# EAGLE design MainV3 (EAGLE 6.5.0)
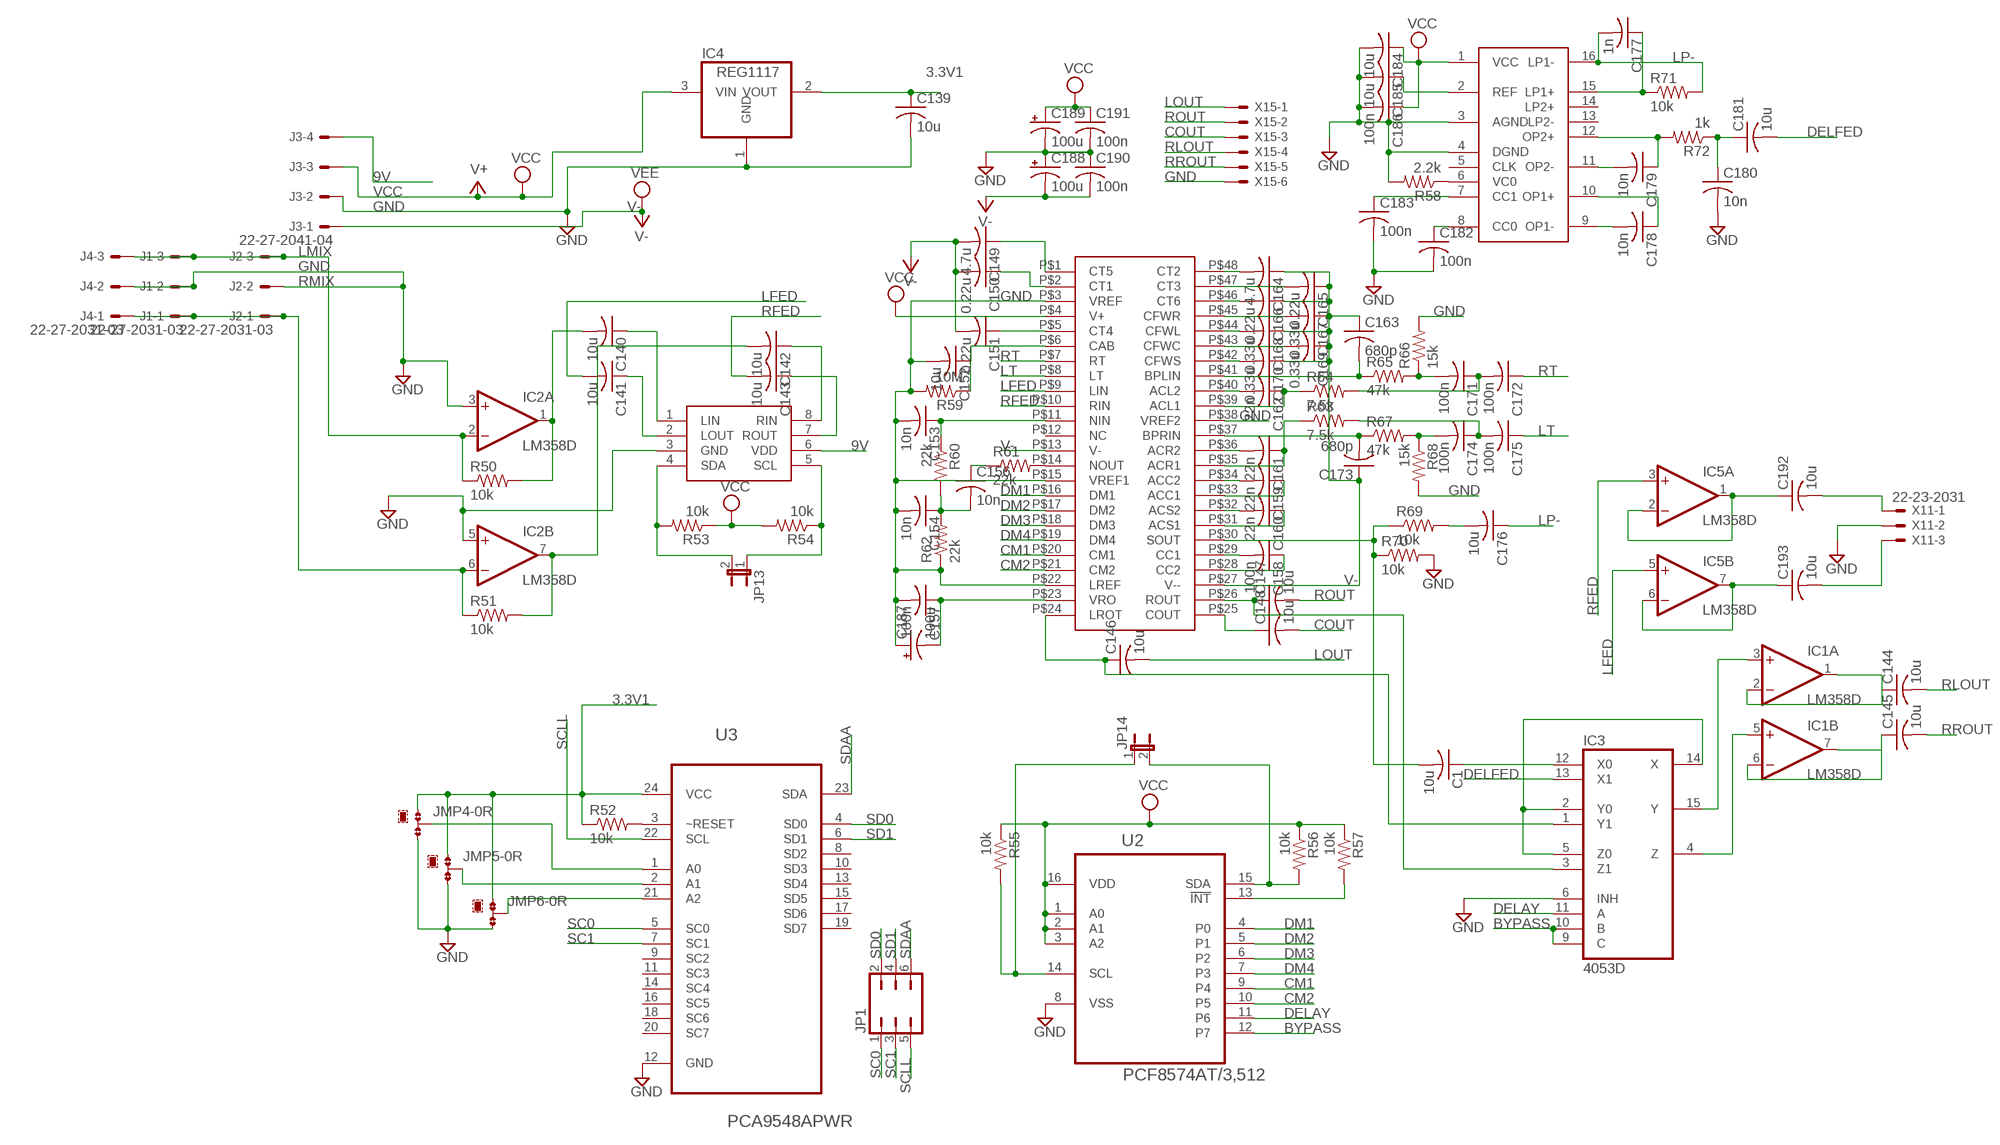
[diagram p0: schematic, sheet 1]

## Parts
C1  10u  C-USC1206  [C1206]
C139  10u  C-USC1206  [C1206]
C140  10u  C-USC1206  [C1206]
C141  10u  C-USC1206  [C1206]
C142  10u  C-USC1206  [C1206]
C143  10u  C-USC1206  [C1206]
C144  10u  C-USC1206  [C1206]
C145  10u  C-USC1206  [C1206]
C146  10u  C-USC1206  [C1206]
C147  10u  C-USC1206  [C1206]
C148  10u  C-USC1206  [C1206]
C149  4.7u  C-USC1206  [C1206]
C150  0.22u  C-USC1206  [C1206]
C151  0.22u  C-USC1206  [C1206]
C152  10u  C-USC1206  [C1206]
C153  10n  C-USC1206  [C1206]
C154  10n  C-USC1206  [C1206]
C156  10n  C-USC1206  [C1206]
C157  100n  C-USC1206  [C1206]
C158  100n  C-USC1206  [C1206]
C159  22n  C-USC1206  [C1206]
C160  22n  C-USC1206  [C1206]
C161  22n  C-USC1206  [C1206]
C162  22n  C-USC1206  [C1206]
C163  680p  C-USC1206  [C1206]
C164  4.7u  C-USC1206  [C1206]
C165  0.22u  C-USC1206  [C1206]
C166  0.22u  C-USC1206  [C1206]
C167  0.33u  C-USC1206  [C1206]
C168  0.33u  C-USC1206  [C1206]
C169  0.33u  C-USC1206  [C1206]
C170  0.33u  C-USC1206  [C1206]
C171  100n  C-USC1206  [C1206]
C172  100n  C-USC1206  [C1206]
C173  680p  C-USC1206  [C1206]
C174  100n  C-USC1206  [C1206]
C175  100n  C-USC1206  [C1206]
C176  10u  C-USC1206  [C1206]
C177  1n  C-USC1206  [C1206]
C178  10n  C-USC1206  [C1206]
C179  10n  C-USC1206  [C1206]
C180  10n  C-USC1206  [C1206]
C181  10u  C-USC1206  [C1206]
C182  100n  C-USC1206  [C1206]
C183  100n  C-USC1206  [C1206]
C184  10u  C-USC1206  [C1206]
C185  10u  C-USC1206  [C1206]
C186  100n  C-USC1206  [C1206]
C187  100u  CPOL-USE2-5  [E2-5]
C188  100u  CPOL-USE2-5  [E2-5]
C189  100u  CPOL-USE2-5  [E2-5]
C190  100n  C-USC1206  [C1206]
C191  100n  C-USC1206  [C1206]
C192  10u  C-USC1206  [C1206]
C193  10u  C-USC1206  [C1206]
IC1  LM358D  [SO08]
IC2  LM358D  [SO08]
IC3  4053D  [SO16]
IC4  REG1117  [SOT223]
IC5  LM358D  [SO08]
J1  22-27-2031-03  [6410-03]
J2  22-27-2031-03  [6410-03]
J3  22-27-2041-04  [6410-04]
J4  22-27-2031-03  [6410-03]
JMP4  0R-JUMPB  [B0R-JMP]
JMP5  0R-JUMPB  [B0R-JMP]
JMP6  0R-JUMPB  [B0R-JMP]
JP1  JP3Q  [JP3Q]
JP13  JP1E  [JP1]
JP14  JP1E  [JP1]
R50  10k  R-US_R1206  [R1206]
R51  10k  R-US_R1206  [R1206]
R52  10k  R-US_R1206  [R1206]
R53  10k  R-US_R1206  [R1206]
R54  10k  R-US_R1206  [R1206]
R55  10k  R-US_R1206  [R1206]
R56  10k  R-US_R1206  [R1206]
R57  10k  R-US_R1206  [R1206]
R58  2.2k  R-US_R1206  [R1206]
R59  10M  R-US_R1206  [R1206]
R60  22k  R-US_R1206  [R1206]
R61  22k  R-US_R1206  [R1206]
R62  22k  R-US_R1206  [R1206]
R63  7.5k  R-US_R1206  [R1206]
R64  7.5k  R-US_R1206  [R1206]
R65  47k  R-US_R1206  [R1206]
R66  15k  R-US_R1206  [R1206]
R67  47k  R-US_R1206  [R1206]
R68  15k  R-US_R1206  [R1206]
R69  10k  R-US_R1206  [R1206]
R70  10k  R-US_R1206  [R1206]
R71  10k  R-US_R1206  [R1206]
R72  1k  R-US_R1206  [R1206]
U2  PCF8574AT/3,512  [SOIC127P1032X265-16N]
U3  PCA9548APWR  [SOP65P640X120-24N]
U$9  SSM2126  [DIP48]
U$10  PT2257  [SO08]
U$11  PT2399  [DIL16]
X11  22-23-2031  [22-23-2031]
X15  22-23-2061  [22-23-2061]

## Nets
3.3V1: C139.1 IC4.2(VOUT) JMP4.1 JMP5.1 JMP6.1 R52.1 U3.24(VCC)
9V: J3.4 U$10.6(VDD)
BYPASS: IC3.9(C) IC3.10(B) U2.12(P7)
CM1: U2.9(P4) U$9.P$20(CM1)
CM2: U2.10(P5) U$9.P$21(CM2)
COUT: C148.2 X15.3
DELAY: IC3.11(A) U2.11(P6)
DELFED: C181.2 IC3.13(X1)
DM1: U2.4(P0) U$9.P$16(DM1)
DM2: U2.5(P1) U$9.P$17(DM2)
DM3: U2.6(P2) U$9.P$18(DM3)
DM4: U2.7(P3) U$9.P$19(DM4)
GND: C139.2 C152.2 C153.2 C154.2 C157.2 C180.2 C182.2 C183.2 C184.2 C185.2 C186.2 C187.+ C188.+ C189.- C190.1 C191.2 IC2.3(A:+IN) IC2.5(B:+IN) IC3.6(INH) IC4.1(GND) J1.2 J2.2 J3.2 J4.2 JMP4.3 JMP5.3 JMP6.3 R58.2 R59.2 R62.1 R66.2 R68.2 R70.2 U2.8(VSS) U3.12(GND) U$9.P$3(VREF) U$9.P$15(VREF1) U$9.P$22(LREF) U$9.P$38(VREF2) U$10.3(GND) U$11.3(AGND) U$11.4(DGND) X11.2 X15.6
LFED: C141.2 IC5.5(B:+IN) U$9.P$9(LIN)
LMIX: IC2.2(A:-IN) J1.3 J2.3 J4.3 R50.1
LOUT: C146.2 X15.1
LP-: C176.1 C177.2 R71.2 U$11.16(LP1-)
LT: C175.1 U$9.P$8(LT)
N$1: C1.1 IC3.12(X0)
N$2: C146.1 IC3.1(Y1) U$9.P$24(LROT)
N$3: C147.1 IC3.3(Z1) U$9.P$26(ROUT)
N$4: C144.1 IC1.1(A:OUT) IC1.2(A:-IN)
N$5: C145.1 IC1.6(B:-IN) IC1.7(B:OUT)
N$7: IC1.3(A:+IN) IC3.15(Y)
N$8: IC1.5(B:+IN) IC3.4(Z)
N$241: C140.2 IC2.1(A:OUT) R50.2
N$242: C192.1 IC5.1(A:OUT) IC5.2(A:-IN)
N$243: C193.1 IC5.6(B:-IN) IC5.7(B:OUT)
N$244: C142.2 IC2.7(B:OUT) R51.2
N$245: C140.1 U$10.1(LIN)
N$246: C142.1 U$10.8(RIN)
N$247: C141.1 U$10.2(LOUT)
N$248: C143.1 U$10.7(ROUT)
N$249: R52.2 U3.3(~RESET)
N$257: C192.2 X11.1
N$258: JMP5.2 U3.2(A1)
N$260: JMP6.2 U3.21(A2)
N$261: JMP4.2 U3.1(A0)
N$262: IC3.2(Y0) IC3.5(Z0) IC3.14(X)
N$263: R57.2 U2.13(!INT)
N$268: C148.1 U$9.P$25(COUT)
N$269: R58.1 U$11.6(VC0)
N$270: C149.1 U$9.P$1(CT5)
N$271: C150.1 U$9.P$2(CT1)
N$272: C151.1 U$9.P$5(CT4)
N$273: C152.1 R59.1 U$9.P$6(CAB)
N$274: R61.2 U$9.P$14(NOUT)
N$278: C153.1 R60.1 U$9.P$11(NIN)
N$279: C193.2 X11.3
N$281: C154.1 C156.2 R60.2 R62.2
N$282: C156.1 R61.1
N$283: C157.1 C187.- U$9.P$23(VRO)
N$284: C158.2 U$9.P$29(CC1)
N$285: C158.1 U$9.P$28(CC2)
N$286: C160.1 U$9.P$31(ACS1)
N$287: C160.2 U$9.P$32(ACS2)
N$289: C159.1 U$9.P$33(ACC1)
N$290: C159.2 U$9.P$34(ACC2)
N$291: C161.1 R63.1 U$9.P$35(ACR1)
N$292: C161.2 U$9.P$36(ACR2)
N$293: C162.2 U$9.P$40(ACL2)
N$294: C162.1 R64.1 U$9.P$39(ACL1)
N$295: C163.2 R65.1 U$9.P$41(BPLIN)
N$296: C166.2 U$9.P$46(CT6)
N$297: C170.2 U$9.P$42(CFWS)
N$298: C169.2 U$9.P$43(CFWC)
N$299: C168.2 U$9.P$44(CFWL)
N$300: C167.2 U$9.P$45(CFWR)
N$301: C165.2 U$9.P$47(CT3)
N$302: C164.2 U$9.P$48(CT2)
N$303: C171.2 R65.2 R66.1
N$304: C171.1 C172.2 R64.2
N$305: C173.2 R67.1 U$9.P$37(BPRIN)
N$306: C174.2 R67.2 R68.1
N$307: C174.1 C175.2 R63.2
N$308: C176.2 R69.2
N$309: C177.1 R71.1 U$11.15(LP1+)
N$310: C178.2 U$11.9(OP1-)
N$311: C179.2 U$11.11(OP2-)
N$312: C178.1 U$11.10(OP1+)
N$313: C179.1 R72.2 U$11.12(OP2+)
N$314: C180.1 C181.1 R72.1
N$315: C183.1 U$11.7(CC1)
N$316: C182.1 U$11.8(CC0)
N$317: C185.1 U$11.2(REF)
N$318: JP13.2 R53.2 U$10.4(SDA)
N$319: JP13.1 R54.1 U$10.5(SCL)
N$320: JP14.2 R56.2 U2.15(SDA)
N$321: JP14.1 R55.2 U2.14(SCL)
RFED: C143.2 IC5.3(A:+IN) U$9.P$10(RIN)
RLOUT: C144.2 X15.4
RMIX: IC2.6(B:-IN) J1.1 J2.1 J4.1 R51.1
ROUT: C147.2 X15.2
RROUT: C145.2 X15.5
RT: C172.1 U$9.P$7(RT)
SC0: JP1.1 U3.5(SC0)
SC1: JP1.3 U3.7(SC1)
SCLL: JP1.5 U3.22(SCL)
SD0: JP1.2 U3.4(SD0)
SD1: JP1.4 U3.6(SD1)
SDAA: JP1.6 U3.23(SDA)
SFED: C1.2 R69.1 R70.1 U$9.P$30(SOUT)
V-: C149.2 C150.2 C151.2 C163.1 C164.1 C165.1 C166.1 C167.1 C168.1 C169.1 C170.1 C173.1 C188.- C190.2 J3.1 U$9.P$13(V-) U$9.P$27(V--) ; supply symbol labelled VEE
VCC: C184.1 C186.1 C189.+ C191.1 IC4.3(VIN) J3.3 R53.1 R54.2 R55.1 R56.1 R57.1 U2.1(A0) U2.2(A1) U2.3(A2) U2.16(VDD) U$9.P$4(V+) U$11.1(VCC) ; supply symbol labelled V+
Unconnected: U3.8(SD2) U3.9(SC2) U3.10(SD3) U3.11(SC3) U3.13(SD4) U3.14(SC4) U3.15(SD5) U3.16(SC5) U3.17(SD6) U3.18(SC6) U3.19(SD7) U3.20(SC7) U$9.P$12(NC) U$11.5(CLK) U$11.13(LP2-) U$11.14(LP2+)

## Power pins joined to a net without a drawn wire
GND: IC3.8(GND)
V+: IC2.8(P:V+)
V-: IC1.4(P:V-) IC2.4(P:V-) IC3.7(VEE) IC5.4(P:V-)
VCC: IC1.8(P:V+) IC3.16(VCC) IC5.8(P:V+)

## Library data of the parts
C1 C139-C154 C156-C186 C190-C193 = adafruit:C-US: CAPACITOR, American symbol
C187-C189 = adafruit:CPOL-US: POLARIZED CAPACITOR, American symbol
IC1 IC2 IC5 = linear:LM358: OP AMP also LM158; LM258; LM2904 Source: http://cache.national.com/ds/LM/LM158.pdf
IC3 = 40xx:4053: Triple 2-channel ANALOG MULTIPLEXER
IC4 = burr-brown:REG1117: 800mA and 1A Low Dropout (LDO) Positive Regulator 1.8V, 2.5V, 2.85V, 3.3V, 5V, and Adj; MPN: REG1117; OC_FARNELL: 1097566; OC_NEWARK: 14P6981
J1 J2 J4 = con-molex:22-?-03: CONNECTOR wire to board 2.54 mm (.1 inch) pitch header; OC_FARNELL: unknown; OC_NEWARK: unknown
J3 = con-molex:22-?-04: CONNECTOR wire to board 2.54 mm (.1 inch) pitch header; OC_FARNELL: unknown; OC_NEWARK: unknown
JMP4-JMP6 = jump-0r-smd:0R-JUMP: SMD 0R 0805 Jumper
JP1 = jumper:JP3Q: JUMPER
JP13 JP14 = jumper:JP1E: JUMPER
R50-R72 = adafruit:R-US_: RESISTOR, American symbol
U2 = PCF8574A:PCF8574AT/3,512: IC, I/O EXPANDER, 8BIT, 16SOIC; MPN: PCF8574AT/3,512; OC_FARNELL: 2101302; OC_NEWARK: 70R6866; PACKAGE: SOIC-16; SUPPLIER: NXP
U3 = PCA9548A:PCA9548APWR: 8-CHANNEL I2C SWITCH WITH RESET; MPN: PCA9548APWR False; OC_FARNELL: 1607855; OC_NEWARK: 22M1602; PACKAGE: TSSOP-24; SUPPLIER: Texas Instruments
U$9 = adafruit:SSM2126
U$10 = adafruit:PT2257
U$11 = adafruit:PT2399
X11 = con-molex:22-23-2031: .100" (2.54mm) Center Header - 3 Pin; MF: MOLEX; MPN: 22-23-2031; OC_FARNELL: 1462950; OC_NEWARK: 30C0862
X15 = con-molex:22-23-2061: .100" (2.54mm) Center Header - 6 Pin; MF: MOLEX; MPN: 22-23-2061; OC_FARNELL: 1462922; OC_NEWARK: 27C1933

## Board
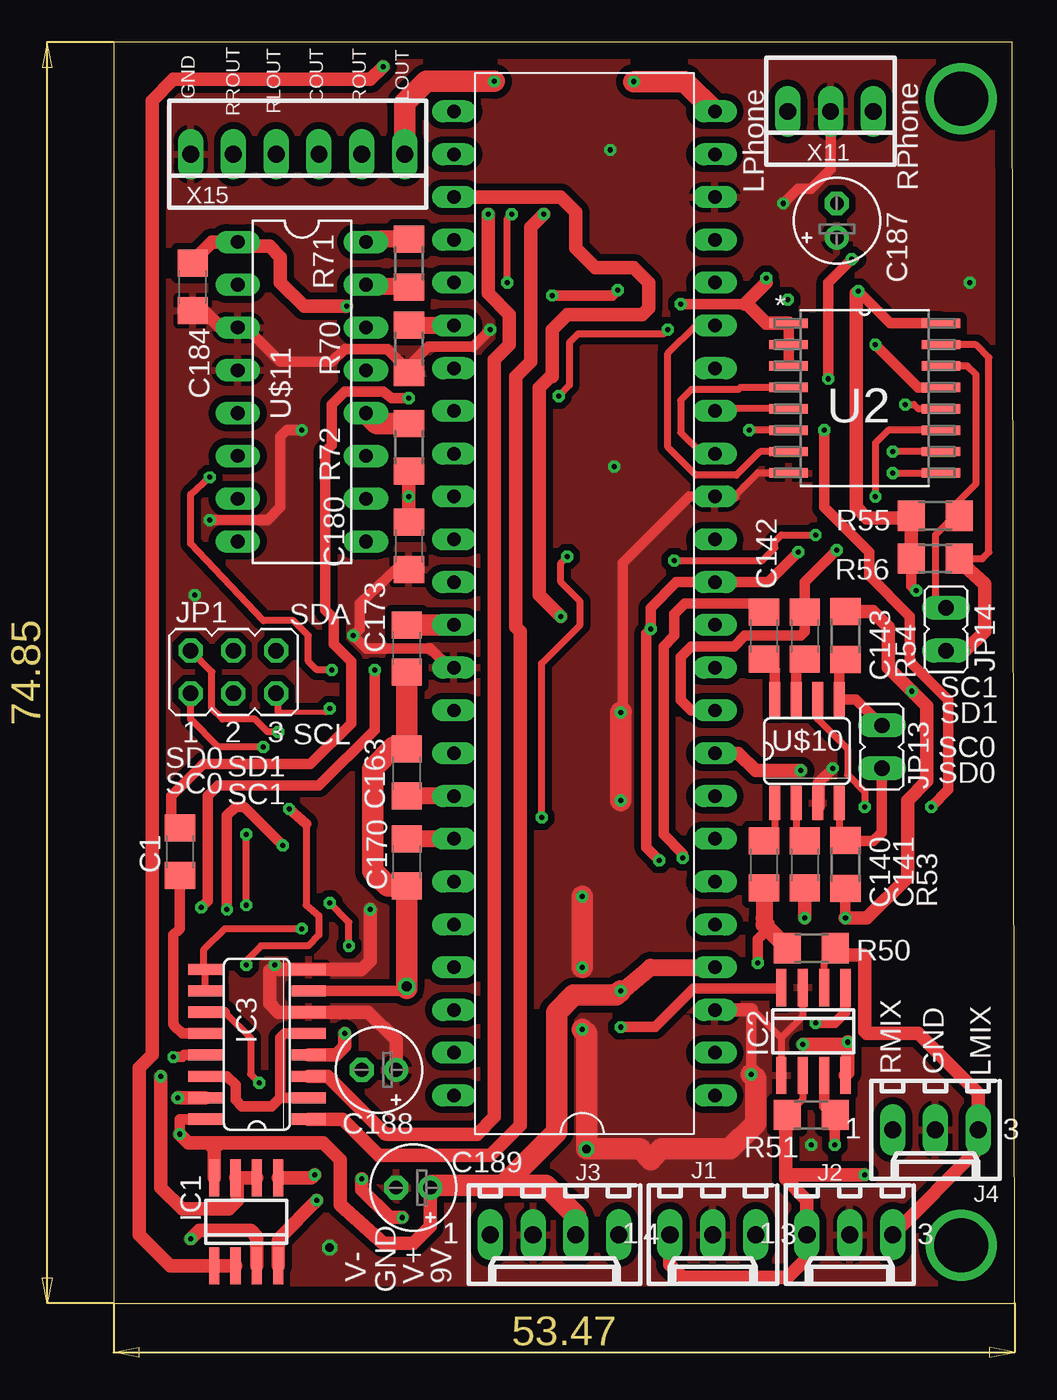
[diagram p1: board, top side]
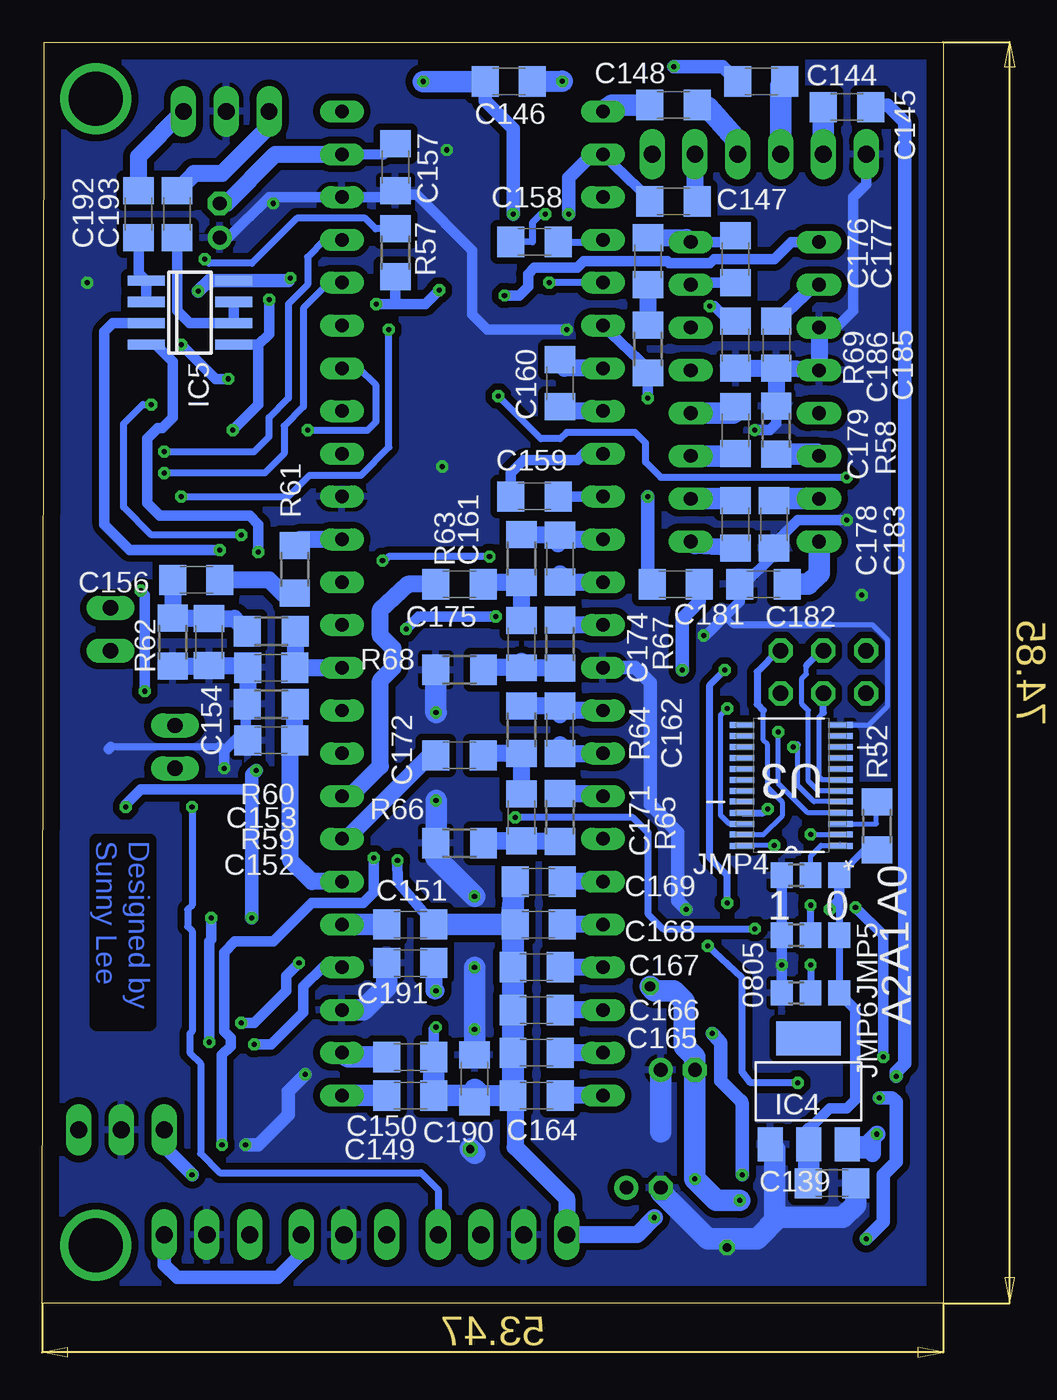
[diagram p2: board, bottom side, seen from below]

Size 57.71 x 78.08 mm. Coordinates in mm from the lower left corner, seen from the top.
Outline: 4.24,3.22 57.71,3.22 57.58,78.08 4.24,78.08 4.24,3.22
Copper layers (1*16): Top 0.035mm / dielectric 1.5mm / Bottom 0.035mm
Design rules "default *": minimum track width 10mil, minimum drill 0.3mm, track to track 6mil, track to pad 6mil, pad to pad 6mil, via to via 6mil, smd to smd 6mil, copper to edge 40mil, drill to drill 8mil, minimum pad ring 10mil, minimum via ring 8mil, stop-mask expansion 4mil, vias tented up to drill 0mil, thermal gap 10mil

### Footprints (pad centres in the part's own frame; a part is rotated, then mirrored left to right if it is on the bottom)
C1206 = smd 1.6 x 1.8: 1 -1.4,0; 2 1.4,0
E2-5 = drill 0.813 pad 1.422: + -1.016,0 | drill 0.813 pad 1.422 octagon: - 1.016,0
SO08 = smd 0.6 x 2.2: 1 -1.905,-2.6; 2 -0.635,-2.6; 3 0.635,-2.6; 4 1.905,-2.6; 5 1.905,2.6; 6 0.635,2.6; 7 -0.635,2.6; 8 -1.905,2.6
SO16 = smd 0.66 x 2.032: 1 -4.445,-3.073; 2 -3.175,-3.073; 3 -1.905,-3.073; 4 -0.635,-3.073; 5 0.635,-3.073; 6 1.905,-3.073; 7 3.175,-3.073; 8 4.445,-3.073; 9 4.445,3.073; 10 3.175,3.073; 11 1.905,3.073; 12 0.635,3.073; 13 -0.635,3.073; 14 -1.905,3.073; 15 -3.175,3.073; 16 -4.445,3.073
SOT223 = smd 1.499 x 2.007: 1 -2.261,-3.15; 2 0.025,-3.15; 3 2.311,-3.15 | smd 3.81 x 2.007: 4 0,3.15
6410-03 = drill 1.016 long: 1 2.54,0; 2 0,0; 3 -2.54,0
6410-04 = drill 1.016 long: 1 3.81,0; 2 1.27,0; 3 -1.27,0; 4 -3.81,0
B0R-JMP = smd 1.5 x 1.3: 1 0,1.7; 2 0,0; 3 0,-1.7
JP3Q = drill 0.914 octagon: 1 -2.54,-1.27; 2 -2.54,1.27; 3 0,-1.27; 4 0,1.27; 5 2.54,-1.27; 6 2.54,1.27
JP1 = drill 0.914 long: 1 0,-1.27; 2 0,1.27
R1206 = smd 1.6 x 1.803: 1 -1.422,0; 2 1.422,0
SOIC127P1032X265-16N = smd 2.286 x 0.559: 1 -4.521,4.445; 2 -4.521,3.175; 3 -4.521,1.905; 4 -4.521,0.635; 5 -4.521,-0.635; 6 -4.521,-1.905; 7 -4.521,-3.175; 8 -4.521,-4.445; 9 4.521,-4.445; 10 4.521,-3.175; 11 4.521,-1.905; 12 4.521,-0.635; 13 4.521,0.635; 14 4.521,1.905; 15 4.521,3.175; 16 4.521,4.445
SOP65P640X120-24N = smd 1.473 x 0.356: 1 -2.921,3.581; 2 -2.921,2.921; 3 -2.921,2.286; 4 -2.921,1.626; 5 -2.921,0.965; 6 -2.921,0.33; 7 -2.921,-0.33; 8 -2.921,-0.965; 9 -2.921,-1.626; 10 -2.921,-2.286; 11 -2.921,-2.921; 12 -2.921,-3.581; 13 2.921,-3.581; 14 2.921,-2.921; 15 2.921,-2.286; 16 2.921,-1.626; 17 2.921,-0.965; 18 2.921,-0.33; 19 2.921,0.33; 20 2.921,0.965; 21 2.921,1.626; 22 2.921,2.286; 23 2.921,2.921; 24 2.921,3.581
DIP48 = drill 0.8 long: P$1 -29.21,-8.89; P$2 -26.67,-8.89; P$3 -24.13,-8.89; P$4 -21.59,-8.89; P$5 -19.05,-8.89; P$6 -16.51,-8.89; P$7 -13.97,-8.89; P$8 -11.43,-8.89; P$9 -8.89,-8.89; P$10 -6.35,-8.89; P$11 -3.81,-8.89; P$12 -1.27,-8.89; P$13 1.27,-8.89; P$14 3.81,-8.89; P$15 6.35,-8.89; P$16 8.89,-8.89; P$17 11.43,-8.89; P$18 13.97,-8.89; P$19 16.51,-8.89; P$20 19.05,-8.89; P$21 21.59,-8.89; P$22 24.13,-8.89; P$23 26.67,-8.89; P$24 29.21,-8.89; P$25 29.21,6.604; P$26 26.67,6.604; P$27 24.13,6.604; P$28 21.59,6.604; P$29 19.05,6.604; P$30 16.51,6.604; P$31 13.97,6.604; P$32 11.43,6.604; P$33 8.89,6.604; P$34 6.35,6.604; P$35 3.81,6.604; P$36 1.27,6.604; P$37 -1.27,6.604; P$38 -3.81,6.604; P$39 -6.35,6.604; P$40 -8.89,6.604; P$41 -11.43,6.604; P$42 -13.97,6.604; P$43 -16.51,6.604; P$44 -19.05,6.604; P$45 -21.59,6.604; P$46 -24.13,6.604; P$47 -26.67,6.604; P$48 -29.21,6.604
SO08' = smd 0.66 x 2.032: 1 -1.905,-3.073; 2 -0.635,-3.073; 3 0.635,-3.073; 4 1.905,-3.073; 5 1.905,3.073; 6 0.635,3.073; 7 -0.635,3.073; 8 -1.905,3.073
DIL16 = drill 0.813 long: 1 -8.89,-3.81; 2 -6.35,-3.81; 3 -3.81,-3.81; 4 -1.27,-3.81; 5 1.27,-3.81; 6 3.81,-3.81; 7 6.35,-3.81; 8 8.89,-3.81; 9 8.89,3.81; 10 6.35,3.81; 11 3.81,3.81; 12 1.27,3.81; 13 -1.27,3.81; 14 -3.81,3.81; 15 -6.35,3.81; 16 -8.89,3.81
22-23-2031 = drill 1 long: 1 -2.54,0; 2 0,0; 3 2.54,0
22-23-2061 = drill 1 long: 1 -6.35,0; 2 -3.81,0; 3 -1.27,0; 4 1.27,0; 5 3.81,0; 6 6.35,0

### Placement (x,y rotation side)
C1  8.17,30.02 90 top
C139  10.84,10.33 0 bottom
C140  42.84,29.26 270 top
C141  45.26,29.26 270 top
C142  42.84,42.84 90 top
C143  45.26,42.84 90 top
C144  15.03,75.74 0 bottom
C145  9.95,74.21 180 bottom
C146  30.02,75.74 0 bottom
C147  20.24,68.63 0 bottom
C148  20.24,74.34 0 bottom
C149  35.86,15.54 0 bottom
C150  35.86,17.83 0 bottom
C151  35.86,25.7 0 bottom
C152  44.12,36.62 180 bottom
C153  44.12,40.94 180 bottom
C154  47.8,42.46 270 bottom
C156  48.56,46.15 180 bottom
C157  36.75,70.66 270 bottom
C158  28.49,66.21 180 bottom
C159  28.49,51.1 0 bottom
C160  26.97,57.83 270 bottom
C161  26.97,47.42 270 bottom
C162  26.97,37.26 270 bottom
C163  21.64,34.72 270 top
C164  28.37,15.54 0 bottom
C165  28.37,18.08 0 bottom
C166  28.37,20.62 0 bottom
C167  28.37,23.16 0 bottom
C168  28.24,25.7 0 bottom
C169  28.24,28.24 0 bottom
C170  21.64,29.38 90 top
C171  29.26,32.05 270 bottom
C172  32.94,35.73 0 bottom
C173  21.64,42.08 90 top
C174  29.26,42.34 270 bottom
C175  32.94,45.89 0 bottom
C176  21.76,65.07 270 bottom
C177  16.56,65.2 90 bottom
C178  16.56,49.45 270 bottom
C179  16.56,55.04 270 bottom
C180  21.76,48.18 270 top
C181  20.11,45.89 0 bottom
C182  14.9,45.89 180 bottom
C183  14.27,49.45 270 bottom
C184  8.94,63.55 270 top
C185  14.14,60.12 270 bottom
C186  16.56,60.12 270 bottom
C187  47.16,67.48 90 top
C188  19.98,17.06 180 top
C189  22.02,10.08 180 top
C190  32.05,16.56 270 bottom
C191  35.86,23.41 180 bottom
C192  51.99,67.86 90 bottom
C193  49.7,67.86 90 bottom
IC1  12.11,8.05 0 top
IC2  45.77,19.35 180 top
IC3  12.75,18.59 90 top
IC4  12.24,15.79 0 bottom
IC5  48.94,62.02 270 bottom
J1  39.8,7.29 180 top
J2  47.92,7.29 180 top
J3  30.4,7.29 180 top
J4  53.01,13.51 180 top
JMP4  12.11,28.62 270 bottom
JMP5  12.11,25.07 270 bottom
JMP6  12.11,21.64 270 bottom
JP1  11.35,40.69 0 top
JP13  49.83,36.24 180 top
JP14  53.64,43.23 180 top
R50  45.64,24.3 180 top
R51  45.64,14.4 0 top
R52  8.17,31.54 90 bottom
R53  47.67,29.26 90 top
R54  47.67,42.84 90 top
R55  53.01,49.96 0 top
R56  53.01,47.42 0 top
R57  36.75,65.58 90 bottom
R58  14.14,55.04 90 bottom
R59  44.12,38.78 180 bottom
R60  44.12,43.1 180 bottom
R61  42.72,46.78 90 bottom
R62  49.96,42.46 90 bottom
R63  29.26,47.42 270 bottom
R64  29.26,37.26 270 bottom
R65  26.97,32.05 270 bottom
R66  32.94,30.53 180 bottom
R67  26.97,42.34 270 bottom
R68  32.94,40.81 180 bottom
R69  21.76,59.86 90 bottom
R70  21.76,59.86 270 top
R71  21.76,64.94 90 top
R72  21.76,54.02 90 top
U2  48.81,56.94 0 top
U3  13.25,33.95 180 bottom
U$9  31.03,44.75 90 top
U$10  PT2257  [SO08']  45.38,35.99 0 top
U$11  15.41,57.32 270 top
X11  46.78,73.96 180 top
X15  15.16,71.42 180 top

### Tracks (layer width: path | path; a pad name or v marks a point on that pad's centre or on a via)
3.3V1  (via drill 0.3)
  Top 0.61: v10.97,26.59 10.97,32.18 11.48,32.69 11.98,32.69 v14.27,30.4
  Bottom 0.305: v14.27,30.4 16.15,30.4 U3.24
  Bottom 0.406: 10.41,27.15 JMP5.1 JMP6.1 | R52.1 8.91,30.12 JMP4.1
  Bottom 0.61: JMP6.1 9.44,20.67 9.44,15.29 9.95,14.78 10.97,14.78 12.21,13.53 | JMP4.1 10.41,27.15 v10.97,26.59
  Bottom 0.813: 12.21,13.53 IC4.2
  Bottom 1.27: IC4.2 12.21,10.36 C139.1
9V  (via drill 0.3)
  Top 0.406: U$10.6 46.02,37.89 47.8,36.11 47.8,34.59 48.81,33.57 v48.81,32.69
  Bottom 0.406: v48.81,32.69 48.81,26.84 49.07,26.59 49.07,25.57 48.81,25.32 48.81,19.35 48.94,19.22 48.94,18.08 48.31,17.45 48.31,12.11 47.16,10.97 35.23,10.97 34.21,9.95 J3.4
BYPASS  (via drill 0.3)
  Top 0.406: IC3.10 IC3.9 | v15.41,25.45 10.84,25.45 9.57,24.18 9.57,23.14 | v29.64,32.05 29.64,41.19 31.92,43.48 31.92,44.88 30.78,46.02 30.78,47.16 v31.16,47.54 | v37.51,47.29 42.72,47.29 43.48,48.05 43.48,48.43 43.86,48.81 v45.89,48.81 | v51.23,56.56 51.73,56.56 51.99,56.31 U2.12
  Top 0.61: 9.57,23.14 IC3.9
  Bottom 0.406: v15.41,25.45 20.87,25.45 21.76,26.34 21.76,31.16 22.65,32.05 v29.64,32.05 | v31.16,47.54 37.13,47.54 37.38,47.29 v37.51,47.29 | v51.23,56.56 51.73,56.56 52.88,55.42 52.88,50.47 51.23,48.81 v45.89,48.81
CM1  (via drill 0.3)
  Top 0.406: v50.46,52.5 U2.9
  Bottom 0.406: U$9.P$20 40.69,63.8 42.21,62.28 42.21,56.43 43.35,55.29 43.35,53.64 44.5,52.5 v50.46,52.5
CM2  (via drill 0.3)
  Top 0.406: U2.10 v50.46,53.77
  Bottom 0.406: v50.46,53.77 45.13,53.77 44.24,54.66 44.24,55.8 43.1,56.94 43.1,62.53 41.96,63.67 41.96,65.32 40.94,66.34 U$9.P$21
COUT
  Bottom 1.27: C148.2 18.21,74.21 16.43,72.18 X15.3
DELAY  (via drill 0.3)
  Top 0.406: 10.84,20.49 12.36,18.97 12.36,16.81 v12.87,16.3 | v18.21,24.43 18.21,25.83 v17.06,26.97 | v17.19,40.81 16.3,40.81 15.79,41.32 15.79,42.84 14.9,43.73 13.13,43.73 8.81,48.31 8.81,51.23 v9.95,52.24 | U2.11 50.21,55.04 49.45,54.28 v49.45,51.1 | v37.13,61.01 36.88,60.75 31.8,60.75 31.29,60.24 31.29,57.7 v30.65,57.07
  Top 0.61: IC3.11 10.84,20.49
  Bottom 0.406: v9.95,52.24 21,52.24 21.89,53.13 21.89,54.28 22.52,54.91 26.59,54.91 26.97,54.53 28.11,54.53 v30.65,57.07 | v12.87,16.3 15.67,16.3 16.17,16.94 16.17,22.52 v18.21,24.43 | v17.06,26.97 17.06,28.62 18.08,29.64 18.08,39.92 v17.19,40.81 | v49.45,51.1 43.1,51.1 41.83,52.37 38.78,52.37 37.13,54.02 v37.13,61.01
DELFED  (via drill 0.3)
  Top 0.61: v19.73,40.81 19.73,37.26 16.43,33.95 10.46,33.95 9.82,33.32 9.82,27.1 v9.44,26.72 | v7.79,17.83 8.3,17.83 8.43,17.95 IC3.13
  Bottom 0.61: C181.2 18.71,45 | v9.44,26.72 7.79,25.07 v7.79,17.83
  Bottom 0.813: 18.71,45 18.71,44.88 19.73,43.86 v19.73,40.81
DM1
  Top 0.406: U2.4 41.45,57.58 41.32,57.45 38.53,57.45 37.89,56.81 37.89,54.91 39.16,53.64 U$9.P$16
DM2
  Top 0.406: U2.5 40.05,56.31 U$9.P$17
DM3  (via drill 0.3)
  Top 0.406: U2.6 v41.96,55.04
  Bottom 0.406: v41.96,55.04 38.4,55.04 37.89,55.55 37.89,57.7 38.91,58.72 U$9.P$18
DM4
  Top 0.406: U2.7 42.59,53.77 41.19,52.37 38.78,52.37 37.13,54.02 37.13,59.61 38.78,61.26 U$9.P$19
GND  (via drill 0.3, 0.5)
  Top 0.406: U$10.3 46.02,32.81 46.15,32.69 | IC2.3 45.13,20.24 43.86,18.97 | 43.86,18.97 IC2.5 | 42.08,20.62 42.21,20.62 43.86,18.97 | U2.8 42.46,52.5 41.07,51.1
  Top 0.61: U$10.3 46.02,34.08 v46.91,34.97 46.15,34.21 46.15,32.69 | v42.08,16.81 42.08,20.62 | 41.07,51.1 U$9.P$15 38.4,51.1 34.46,47.16 34.46,38.4 v34.34,38.27 | v26.59,61.01 25.57,59.99 22.91,59.99 21.76,58.85 R70.2 21.76,58.59 20.49,59.86 17.95,59.86 17.19,59.1 14.14,59.1 12.11,61.13 | 13.51,22.98 v13.81,23.29 | IC3.8 15.29,23.03 | C180.2 21,46.78 18.84,44.75 18.84,43.23 v18.46,42.84 19.22,42.08 23.03,42.08 24.18,40.94 U$9.P$38 | v15.41,55.04 14.52,55.04 14.14,54.66 14.14,50.47 13.38,49.7 v9.95,49.7 | X11.2 46.78,70.53 45.64,69.39 44.88,69.39 v43.99,68.5
  Top 0.813: U$9.P$3 42.08,20.62 | C184.2 9.57,62.15 10.59,61.13 U$11.3 | 13.51,22.98 13.51,21 14.02,20.49 IC3.6 19.35,20.49 21,18.84 C188.+ | v13.81,23.29 14.06,23.03 15.29,23.03 18.97,23.03 19.48,23.54 v19.48,26.59
  Top 1.016: 12.11,61.13 U$11.3
  Top 1.27: v32.05,27.35 v32.05,23.16 | v34.34,33.07 v34.34,38.27 34.36,38.3 | v32.05,19.48 32.3,19.22 v32.3,12.37 35.48,12.37 36.11,11.73 36.75,12.37 40.81,12.37 42.34,13.89 42.34,16.56 v42.08,16.81
  Bottom 0.305: U3.12 8.66,37.54 7.54,38.65 7.54,42.59 8.43,43.48 10.97,43.48
  Bottom 0.406: 10.97,43.48 16.68,43.48 17.19,43.99 | 47.16,36.24 53.64,36.24 | v43.99,68.5 43.61,68.88
  Bottom 0.61: 46.91,35.99 46.15,36.75 45.64,36.75 C152.2 45.64,36.75 45.64,41.06 | JMP6.3 v13.81,23.29 JMP5.3 JMP4.3 | v18.46,42.84 18.33,42.84 17.19,43.99 16.3,44.88 C182.2 16.05,45.89 14.4,47.54 14.4,48.05 C183.2 14.14,48.18 14.14,48.43 12.87,49.7 v9.95,49.7 | R58.2 14.14,55.42 14.52,55.04 v15.41,55.04 | X15.6 8.81,69.64 9.57,68.88 9.57,62.15 10.59,61.13 U$11.3 | C187.+ 46.66,66.47 44.24,68.88 43.61,68.88 U$9.P$22 37.27,68.88 C157.2 37.12,69.01 35.48,69.01 32.18,65.7 32.18,61.89 31.29,61.01 v26.59,61.01 | v46.91,34.97 46.91,35.99 | 46.91,35.99 47.16,36.24 | 53.64,36.24 53.77,36.11
  Bottom 0.813: U$9.P$38 22.52,40.94 21.64,40.05 21.64,32.81 19.98,31.16 19.98,27.1 v19.48,26.59 | v45.64,12.62 44.88,12.62 43.1,14.4 43.1,15.79 v42.08,16.81
  Bottom 1.016: R62.1 47.82,41.04 C154.2 45.64,41.06 C153.2 45.52,38.8 R59.2 | C186.2 C185.2 | C185.2 R58.2 | C185.2 U$11.4 U$11.3
  Bottom 1.27: C139.2 9.44,9.07 10.21,8.3 14.02,8.3 | IC4.1 14.27,12.37 14.24,12.34 14.24,8.53 14.02,8.3 | C191.2 37.26,22.01 38.65,20.62 U$9.P$3 | v32.05,23.16 v32.05,19.48 C190.1 | v32.05,27.35 34.36,29.66 R66.2 34.34,30.55 v34.34,33.07 | R68.2 34.36,38.3 v34.34,38.27 | C189.- 21,9.82 18.21,7.03 15.29,7.03 14.02,8.3 | C188.+ 21,13.38 | 32.05,12.11 v32.3,12.37
  other vias: 33.95,52.88 55.04,63.8 33.7,71.67 9.06,45.26 17.06,6.52
  pour Top (isolate 0.406): 4.74,77.52 54.02,77.52 57.07,74.47 57.07,3.86 4.74,3.86
  pour Bottom (isolate 0.406): 5,77.52 57.07,77.52 57.07,3.86 4.74,3.86 4.74,77.52
LFED  (via drill 0.3)
  Top 0.61: v46.4,55.04 46.4,50.47 49.07,47.8 49.07,46.4 51.48,43.99 51.48,41.32 53.77,39.03 53.77,33.7 v52.75,32.69
  Top 0.813: C141.2 v45.26,26.08 | v45,34.84 42.34,34.84 41.32,35.86 U$9.P$9
  Bottom 0.61: IC5.5 44.88,60.12 | 44.88,60.12 44.24,60.75 v44.24,62.78 | 44.88,60.12 44.88,56.56 v46.4,55.04 | v52.75,32.69 52.75,32.81 51.86,33.7 45.64,33.7 45.26,33.32
  Bottom 0.813: v45.26,26.08 45.26,33.32 45.26,34.59 v45,34.84
LMIX
  Top 0.406: IC2.2 46.4,23.41 46.66,23.67 46.66,23.9 R50.1
  Top 0.813: 46.66,23.9 48.71,23.9 48.81,23.8 48.81,19.35 48.94,19.22 51.99,19.22 55.55,15.67 J4.3 55.55,12.37 J2.3 50.46,7.67 50.21,7.92
  Bottom 0.813: J1.3 42.34,6.14 43.73,4.75 49.7,4.75 50.46,5.51 J2.3
LOUT  (via drill 0.3)
  Top 1.27: v26.84,75.74 22.78,75.74 21.51,74.47 X15.1
  Bottom 1.27: C146.2 v26.84,75.74
LP-
  Top 1.016: R71.2 19.25,66.36 U$11.16
  Bottom 0.61: U$11.16 16.94,66.21 C177.2
  Bottom 1.016: C176.1 19.48,66.47 U$11.16
LT
  Bottom 1.016: U$9.P$8 39.42,33.32 37.64,35.1 37.64,40.18 36.88,40.94 36.88,42.08 37.64,42.84 37.64,44.37 35.99,45.89 C175.1
N$1
  Top 0.61: C1.1 8.17,25.55 arc-45 8.1,25.37 7.79,25.07 7.79,19.84 arc45 7.87,19.66 8.3,19.22 IC3.12
N$2  (via drill 0.3)
  Top 0.813: v29.76,67.86 29,67.1 29,59.1 28.11,58.21 28.11,43.35 28.37,43.1 28.37,13.76 26.59,11.98 19.98,11.98 17.83,14.14 IC3.1
  Top 1.27: v35.1,75.74 38.15,75.74 U$9.P$24
  Bottom 0.813: C146.1 31.42,74.6 31.16,74.34 30.02,73.2 29.76,72.94 v29.76,67.86
  Bottom 1.27: C146.1 v35.1,75.74
N$3  (via drill 0.3)
  Top 0.813: v26.46,67.86 26.46,63.17 27.73,61.89 27.73,60.12 26.84,59.23 26.84,14.27 25.83,13.25 20.47,13.25 arc-45 20.29,13.33 16.94,16.68 IC3.3
  Bottom 0.61: C147.1 21.64,68.76 U$9.P$26 25.07,71.42
  Bottom 0.813: v26.46,67.86 26.46,70.02 25.07,71.42
N$4  (via drill 0.3)
  Top 0.813: IC1.2 IC1.1 7.6,5.45 5.76,7.29 5.76,17.19 6.52,17.95 6.52,74.59 7.79,75.87 19.48,75.87 v20.24,76.63
  Bottom 0.813: v20.24,76.63 17.32,76.63 C144.1
N$5  (via drill 0.3)
  Top 0.813: IC1.6 IC1.7 arc-45 11.59,10.6 11.59,9.3 11.09,8.81 8.3,8.81 7.03,10.08 v7.03,16.68
  Bottom 0.813: v7.03,16.68 7.03,16.94 6.52,17.45 6.52,73.33 7.54,74.34 8.43,74.34 C145.1
N$6  (via drill 3.2)
  other vias: 54.53,6.65
N$7  (via drill 0.3)
  Top 0.813: IC1.3 12.75,7.16 12.36,7.54 9.32,7.54 v8.81,7.03 | v8.05,15.41 IC3.15
  Bottom 0.813: v8.81,7.03 7.79,8.05 7.79,10.84 7.03,11.6 7.03,15.16 7.29,15.41 v8.05,15.41
N$8  (via drill 0.3)
  Top 0.813: IC1.5 15.88,10.65 arc45 16.05,10.72 v16.17,10.84 | v17.95,19.22 17.95,18.57 arc-45 17.88,18.39 17.45,17.95 IC3.4
  Bottom 0.813: v16.17,10.84 16.17,15.05 arc-45 16.25,15.23 17.45,16.43 17.45,18.61 arc-45 17.52,18.79 v17.95,19.22
N$9  (via drill 3.2)
  other vias: 54.53,74.72
N$241  (via drill 0.3)
  Top 0.61: IC2.1 47.67,20.49 47.04,19.86 v45.89,19.86 | 43.15,25.37 43.15,25.78 42.84,26.08 | v42.46,23.41 42.46,24.81 43.09,25.43
  Top 1.016: C140.2 42.84,26.08 42.84,25.68 43.09,25.43 43.15,25.37 R50.2
  Bottom 0.61: v45.89,19.86 45.13,19.86 43.23,21.76 43.23,22.65 v42.46,23.41
N$242
  Bottom 0.61: IC5.2 IC5.1 51.99,64.38 C192.1
N$243
  Bottom 0.61: C193.1 49.7,62.15 48.94,61.39 IC5.6 IC5.7
N$244  (via drill 0.3)
  Top 0.406: IC2.7 46.4,15.06 R51.2
  Top 0.61: IC2.7 46.4,14.91 47.04,14.27 v47.04,12.62 | v38.02,29.64 38.02,29.89 36.88,31.03 36.88,42.21 37.51,42.84 37.51,44.11 38.15,44.75 42.34,44.75 C142.2
  Bottom 0.61: v47.04,12.62 47.04,17.95 46.53,18.46 46.53,18.97 46.91,19.35 46.91,24.05 46.27,24.68 43.99,24.68 41.7,26.97 38.65,26.97 38.02,27.61 v38.02,29.64
N$245
  Top 0.406: U$10.1 43.48,31.04 C140.1
N$246
  Top 0.61: U$10.8 43.48,40.81 C142.1
N$247
  Top 0.406: U$10.2 44.75,31.16 C141.1
N$248
  Top 0.61: U$10.7 44.75,40.94 C143.1
N$249
  Bottom 0.305: U3.3 8.2,31.67 R52.2
N$257
  Bottom 1.016: C192.2 51.99,71.29 X11.1
N$258  (via drill 0.3)
  Top 0.406: v12.11,26.84 v12.11,31.03
  Bottom 0.305: v12.11,31.03 U3.2
  Bottom 0.406: JMP5.2 v12.11,26.84
N$260  (via drill 0.3)
  Top 0.406: 15.67,31.67 15.67,26.84 16.43,26.21 16.43,25.07 15.79,24.43 13,24.43 12.11,23.54 v12.11,23.29
  Top 0.61: 15.67,31.67 v14.65,32.56
  Bottom 0.406: U3.21 14.93,32.33 v14.65,32.56 | v12.11,23.29 JMP6.2
N$261
  Bottom 0.305: JMP4.2 12.11,29.76 11.48,30.4 10.36,30.4
  Bottom 0.406: 10.36,30.4 U3.1
N$262
  Top 0.61: IC3.2 14.14,15.41 | IC3.5 14.4,19.22 14.14,18.97 14.14,15.41 | 14.14,15.41 13.63,14.91 11.86,14.91 11.48,15.29 11.48,16.18 10.97,16.68 IC3.14
N$263  (via drill 0.3)
  Top 0.406: v48.05,65.2 48.31,65.2
  Top 0.61: U2.13 51.99,57.58 v49.45,60.12 | v46.66,58.08 46.66,63.8 v48.05,65.2
  Bottom 0.406: R57.2 37.92,67 38.53,67.61 42.59,67.61 45.26,64.94 47.8,64.94 v48.05,65.2
  Bottom 0.61: v49.45,60.12 47.42,58.08 v46.66,58.08
N$268
  Bottom 1.27: C148.1 23.92,74.34 U$9.P$25
N$269
  Bottom 1.27: R58.1 11.75,53.61 U$11.6
N$270
  Bottom 1.27: C149.1 U$9.P$1
N$271
  Bottom 1.27: C150.1 39.54,17.83 U$9.P$2
N$272
  Bottom 1.27: C151.1 U$9.P$5
N$273
  Bottom 1.016: R59.1 42.71,38.76 C152.1 42.97,36.36 42.97,29.51 41.7,28.24 U$9.P$6
N$274
  Bottom 1.016: U$9.P$14 42.36,48.56 R61.2
N$278
  Bottom 1.016: R60.1 42.69,40.96 C153.1 U$9.P$11
N$279
  Bottom 1.016: 49.7,69.52 C193.2 48.69,70.28 47.04,70.28 44.24,73.07 X11.3
N$281
  Bottom 1.016: C156.2 R62.2 47.82,43.89 C154.1 46.3,43.86 R60.2
N$282
  Bottom 1.016: R61.1 43.45,45.36 44.24,46.15 C156.1
N$283
  Bottom 0.61: C157.1 37.5,71.41 U$9.P$23
  Bottom 1.016: C187.- 46.78,68.5 43.86,71.42 U$9.P$23
N$284  (via drill 0.3)
  Top 0.406: v27.61,63.8 27.61,67.61 v27.86,67.86
  Bottom 0.406: U$9.P$29 v27.61,63.8 | v27.86,67.86 28.11,67.86 28.62,67.36 28.62,66.23 C158.2
N$285
  Bottom 0.406: C158.1 24.94,66.21 U$9.P$28
N$286
  Bottom 1.016: U$9.P$31 26.71,58.72 C160.1
N$287
  Bottom 1.016: U$9.P$32 26.97,56.18 C160.2
N$289
  Bottom 0.61: U$9.P$33 25.57,53.64 25.95,53.26 29.13,53.26 29.89,52.48 C159.1
N$290
  Bottom 0.61: U$9.P$34 C159.2
N$291
  Bottom 1.016: U$9.P$35 26.71,48.56 C161.1 27.08,48.29 27.61,48.81 29.23,48.82 R63.1
N$292
  Bottom 1.016: C161.2 26.97,46.53 26.46,46.02 24.31,46.02 U$9.P$36
N$293
  Bottom 1.016: C162.2 26.97,36.37 26.46,35.86 24.31,35.86 U$9.P$40
N$294
  Bottom 1.016: U$9.P$39 26.71,38.4 C162.1 26.97,38.15 27.48,38.65 29.23,38.66 R64.1
N$295
  Top 1.016: U$9.P$41 C163.2
  Bottom 1.016: R65.1 24.45,33.47 U$9.P$41
N$296
  Bottom 1.016: U$9.P$46 C166.2
N$297
  Top 1.016: U$9.P$42 C170.2
N$298
  Bottom 1.016: U$9.P$43 C169.2
N$299
  Bottom 1.016: U$9.P$44 C168.2
N$300
  Bottom 1.016: U$9.P$45 C167.2
N$301
  Bottom 1.016: U$9.P$47 C165.2
N$302
  Bottom 1.016: U$9.P$48 C164.2
N$303
  Bottom 1.016: R65.2 31.03,30.63 | 31.03,30.63 31.41,30.63 R66.1 31.39,30.65 | C171.2 31.02,30.64 31.03,30.63
N$304
  Bottom 1.016: C171.1 R64.2 31.01,35.83 31.03,35.86 31.41,35.86 C172.2
N$305
  Top 1.27: U$9.P$37 C173.2
  Bottom 1.016: U$9.P$37 26.69,43.48 R67.1
N$306
  Bottom 1.016: R67.2 29.23,40.92 C174.2 29.26,41.32 29.64,40.94 31.39,40.94 R68.1
N$307
  Bottom 1.016: C174.1 R63.2 30.8,46 C175.2
N$308
  Bottom 1.016: C176.2 R69.2
N$309
  Top 1.016: R71.1 21.91,63.65 22.02,63.55 19.35,63.55 U$11.15
  Bottom 0.61: C177.1 19.1,63.8 U$11.15
N$310
  Bottom 1.016: C178.2 18.97,48.18 U$11.9
N$311
  Bottom 1.27: U$11.11 16.69,53.51 C179.2
N$312
  Bottom 1.27: U$11.10 16.56,50.97 C178.1
N$313
  Top 1.27: R72.2 19.86,55.42 19.25,56.03 19.25,56.08 U$11.12
  Bottom 1.27: U$11.12 16.69,56.05 C179.1
N$314  (via drill 0.3)
  Top 0.813: R72.1 v21.76,51.1 C180.1
  Bottom 0.813: v21.76,51.1 21.76,46.14 C181.1
N$315
  Bottom 1.27: U$11.7 14.27,50.97 C183.1
N$316
  Bottom 1.27: U$11.8 11.6,46.53 12.24,45.89 C182.1
N$317
  Bottom 0.813: U$11.2 11.86,63.67 C185.1
N$318
  Top 0.406: U$10.4 47.29,30.8 R53.2
  Top 0.61: JP13.2 49.83,31.16 49.32,30.65 47.7,30.65 R53.2
N$319
  Top 0.61: R54.1 47.29,41.04 U$10.5 48.28,39.06 JP13.1
N$320
  Top 0.406: R56.2 55.8,47.42 56.18,47.8 56.18,59.36 55.42,60.12 U2.15
  Top 0.813: R56.2 54.43,47.27 55.93,45.89 55.93,43.1 54.78,41.96 JP14.2
N$321
  Top 0.406: R55.2 54.15,49.96 | 54.15,49.96 53.01,48.81 53.01,45.13 JP14.1 | 54.15,49.96 54.15,50.59 55.42,51.86 55.42,58.34 54.91,58.85 U2.14
RFED  (via drill 0.3)
  Top 0.61: U$9.P$10 38.53,38.4 37.89,39.03 37.89,41.58 38.53,42.21 41.07,42.21 41.7,42.84 45,42.84 45.26,43.1 C143.2 45.26,46.02 v47.16,47.92
  Bottom 0.61: v47.16,47.92 52.5,47.92 54.02,49.45 54.02,60.88 53.51,61.39 IC5.3
RLOUT
  Bottom 1.27: X15.4 13.89,75.48 C144.2
RMIX  (via drill 0.3)
  Top 0.406: IC2.6 45.13,15.31 R51.1
  Top 0.813: 44.12,10.84 44.12,10.59 45.38,9.32 J2.1 45.38,5.89 44.24,4.75 38.02,4.75 37.26,5.51 J1.1 | 44.12,10.84 44.12,14.29 R51.1 | v48.81,10.84 44.12,10.84
  Bottom 0.813: J4.1 50.46,12.49 v48.81,10.84
ROUT
  Bottom 1.016: X15.2 18.97,68.76 C147.2
RROUT
  Bottom 1.27: X15.5 C145.2
RT
  Bottom 1.016: U$9.P$7 39.67,30.78 34.72,35.73 C172.1
SC0  (via drill 0.3)
  Top 0.406: v13.13,36.24 10.46,36.24 8.81,37.89 JP1.1
  Bottom 0.305: U3.5 11.91,32.99 12.87,33.95 12.87,36.37
  Bottom 0.406: 12.87,36.37 v13.13,36.24
SC1
  Bottom 0.305: U3.7 11.43,34.28 11.6,34.46 11.6,38.02 11.35,38.27
  Bottom 0.406: 11.35,38.27 JP1.3
SCLL  (via drill 0.3)
  Top 0.305: v17.06,38.53 16.81,38.27 14.02,38.27
  Top 0.406: 14.02,38.27 14.02,39.29 JP1.5
  Bottom 0.305: U3.22 16.94,31.67 17.45,32.18 17.45,38.15 v17.06,38.53
SD0  (via drill 0.3)
  Top 0.305: v14.02,37.13 13.89,37.13
  Top 0.406: 13.89,37.13 13.38,37.13 12.62,37.89 10.71,37.89 10.08,38.53 10.08,40.69 JP1.2
  Bottom 0.305: U3.4 12.26,32.33 14.02,34.08 v14.02,37.13
SD1
  Bottom 0.305: U3.6 11.65,33.62 12.24,34.21 12.24,38.4 12.62,38.78 12.62,40.31 12.36,40.56 12.36,41.07
  Bottom 0.406: JP1.4 11.48,41.96 12.36,41.07
SDAA
  Bottom 0.305: U3.23 14.9,31.03 13.76,32.18 13.76,32.94 14.65,33.83 14.65,36.37 14.9,36.62 14.9,38.4
  Bottom 0.406: JP1.6 14.02,41.96 15.29,40.69 15.29,38.78 14.9,38.4
SFED  (via drill 0.3 pad 0.25)
  Top 0.61: v21.76,56.94 20.75,56.94 20.24,57.32 17.95,57.32 17.19,56.56 17.19,54.15 16.81,53.77 16.81,44.37 17.32,43.86 17.32,42.34 18.33,41.32 18.33,37.64 15.92,35.23 9.57,35.23 7.67,33.32 7.67,31.93 C1.2
  Top 1.016: R70.1 24.28,61.28 U$9.P$30
  Bottom 0.61: U$9.P$30 21.76,58.72 R69.1 v21.76,56.94
V-  (via drill 0.3, 0.6)
  Top 0.61: IC3.7 21.51,21.76 21.64,21.89 | v36.62,29.51 35.86,30.27 35.86,42.97 v36.11,43.23 36.11,44.5 37.64,46.02 U$9.P$13 43.1,46.02 v44.88,47.8 | v34.34,19.6 36.37,19.6 38.65,21.89 43.8,21.89 IC2.4
  Top 0.813: U$9.P$27 30.78,68.88 31.67,67.99 31.67,65.83 32.81,64.69 35.1,64.69 35.99,63.8 35.99,62.28 35.61,61.89 31.16,61.89 30.27,61.01 30.27,58.21 30.14,58.21 29.51,57.58 29.51,45.26 v30.78,43.99 | v18.97,10.59 18.97,9.95 20.62,8.3 v21.38,8.3 | IC1.4 14.02,6.67 arc-45 14.09,7.11 v16.3,9.32
  Top 1.27: C173.1 C163.1 21.51,36.24 20.87,36.24 19.6,34.97 19.6,28.88 20.5,27.98 C170.1 v21.64,22.02 21.64,21.89
  Bottom 0.61: C151.2 36.62,28.24 v36.62,29.51 | v34.34,19.6 34.46,19.48 C150.2 | v30.78,43.99 35.35,43.99 v36.11,43.23 | IC5.4 50.97,60.12 49.96,59.1 49.96,55.8 50.59,55.16 50.85,55.16 51.48,54.53 51.48,50.72 50.72,49.96 45.38,49.96 44.88,49.45 v44.88,47.8
  Bottom 1.016: v21.38,8.3 22.4,7.29 J3.1 26.59,9.44 29.64,12.5 C168.1 C169.1
  Bottom 1.27: C164.1 31.67,15.54 32.05,15.92 C190.2 32.05,15.54 C149.2 C150.2 | C164.1 C165.1 C166.1 C167.1 29.77,25.57 C168.1 C151.2 | C169.1 29.89,25.7 29.76,25.95 29.76,25.57 | C164.1 | v21.64,22.02 21.38,21.76 20.24,21.76 19.6,21.13 19.6,18.46 18.97,17.83 C188.- v18.97,10.59 17.7,9.32 v16.3,9.32
VCC  (via drill 0.3, 0.3 pad 0.2)
  Top 0.406: v42.97,64.05 42.97,63.8
  Top 0.61: v30.27,63.04 33.83,63.04 v34.14,63.36 | IC3.16 8.17,14.14 v8.17,13.25 | 11.86,65.96 U$11.1 | R53.1 v47.67,26.08 | U2.3 U2.2 U2.1 | U2.16 50.34,61.39 v48.43,63.29 48.31,63.17 | 41.83,62.53 41.7,62.53 v37.89,62.53 | R56.1 51.58,45.79 v51.86,45.51
  Top 0.813: C184.1 8.94,65.07 10.08,66.21 U$11.1 | v18.08,62.4 15.54,62.4 14.14,63.8 14.14,65.32 13.51,65.96 11.86,65.96 | R54.2 49.3,44.27 50.21,43.35 50.21,40.94 v51.61,39.54 52.5,38.65 52.5,34.21 51.35,33.07 51.35,28.49 48.94,26.08 v47.67,26.08 | C189.+ 23.03,7.79 22.02,6.78 20.24,6.78 17.7,9.06 17.7,11.73 16.68,12.75 10.59,12.75 | 10.59,12.75 8.68,12.75 v8.17,13.25 | 48.31,63.17 48.31,50.47 48.94,49.83 51.46,49.83 R55.1 R56.1 | U2.1 42.97,61.39 41.83,62.53 | 42.97,63.8 41.7,62.53 | v45.13,18.59 47.67,18.59 v47.8,18.71 47.8,16.88 IC2.8 | IC1.8 10.21,12.26 arc45 10.13,12.44 IC4.3 10.38,12.64 arc45 10.56,12.72 10.59,12.75
  Top 1.016: v34.34,21.76 34.46,21.76 36.11,23.16 U$9.P$4
  Top 1.27: v34.34,21.76 34.08,21.51 31.54,21.51 30.53,20.49 30.53,13.38 27.41,10.27 | C189.+ 23.16,10.21 27.35,10.21 27.41,10.27 | J3.3 31.67,8.43 29.89,10.21 27.48,10.21 27.41,10.27
  Bottom 0.406: 43.1,63.93 v42.97,64.05
  Bottom 0.61: U$11.1 13.25,66.21 14.27,65.2 17.83,65.2 18.08,64.94 20.49,64.94 20.62,65.07 25.57,65.07 25.95,64.69 28.49,64.69 28.88,64.31 28.88,63.55 29.38,63.04 v30.27,63.04 | 16.56,61.64 17.06,61.64 17.83,62.4 v18.08,62.4 | v45.13,18.59 44.12,18.59 42.21,20.49 42.21,22.02 41.07,23.16 U$9.P$4 | v47.67,26.08 47.67,24.81 47.8,24.68 v47.8,18.71 | 8.43,12.11 9.39,12.11 | v37.89,62.53 36.88,62.53 | 36.88,62.53 34.97,62.53 v34.14,63.36 | R57.1 36.75,62.66 36.88,62.53 | v51.86,45.51 51.61,45.26 v51.61,39.54
  Bottom 0.813: C186.1 16.56,61.64 | v48.43,63.29 47.8,63.93 IC5.8 43.1,63.93
  Bottom 1.016: C191.1 34.46,22.65 34.46,21.76 v34.34,21.76 | IC4.3 8.78,12.64 v8.17,13.25 8.43,13 8.43,12.11

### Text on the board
Bottom: Designed by / Sunny Lee
tPlace: GND | COUT | ROUT | LOUT | RROUT | RLOUT | LPhone | RPhone | SDA | SC1 | SCL | SD1 | SC0 | SD0 | SD1 | SC0 | SD0 | SC1 | LMIX | RMIX | GND | V- | V+ | 9V | GND
bPlace: A0 | 1 0 | A1 | A2 | 0805
_tNames: C27 | C28 | C30 | C29 | C35 | C34 | C33 | C32 | C36 | C37 | R11 | X2 | C38 | R12 | C8 | C9 | C11 | C10 | C16 | C15 | C14 | C13 | C39 | IC2 | C17 | C18 | R5 | X1 | C19 | R6 | C40 | X10 | X11 | X9 | X12
_bNames: IC1 | R10 | R9 | C31 | C26 | R7 | R8 | C21 | C25 | C24 | C20 | C22 | R4 | R3 | C23 | C12 | C7 | R1 | R2 | C2 | C1 | C6 | C5 | C4 | C3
